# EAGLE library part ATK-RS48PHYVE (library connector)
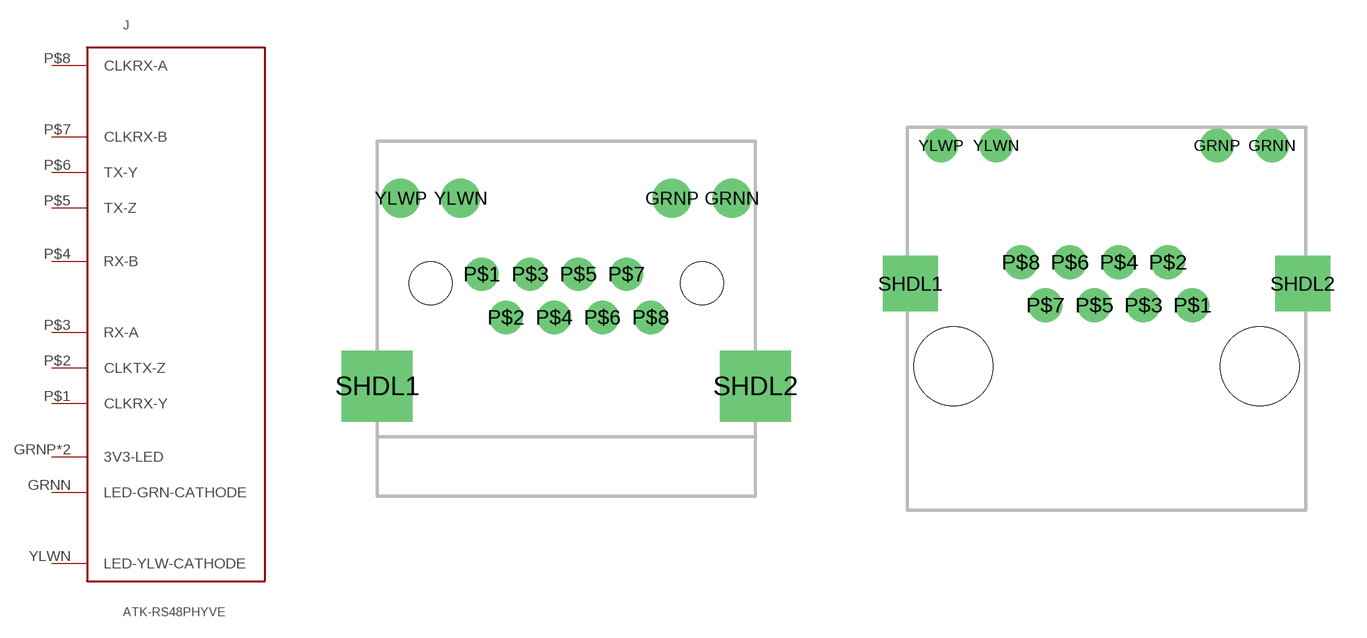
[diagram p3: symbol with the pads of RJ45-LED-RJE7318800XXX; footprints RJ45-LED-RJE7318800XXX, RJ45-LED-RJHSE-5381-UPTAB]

Designator prefix J

## ATK-RS48PHYVERJ45LED  [RJ45-LED-RJE7318800XXX]
GRNN  LED-GRN-CATHODE
GRNP  3V3-LED
P$1  CLKRX-Y
P$2  CLKTX-Z
P$3  RX-A
P$4  RX-B
P$5  TX-Z
P$6  TX-Y
P$7  CLKRX-B
P$8  CLKRX-A
YLWN  LED-YLW-CATHODE
YLWP  3V3-LED

## ATK-RS48PHYVERJ45LEDTABUP  [RJ45-LED-RJHSE-5381-UPTAB]
Pads as for RJ45-LED-RJE7318800XXX

## ATK-RS48PHYVERJ45TABUPSMD  [RJ45-LED-SMD-RJWURTH-634008137521]
Pads as for RJ45-LED-RJE7318800XXX

## Footprint RJ45-LED-RJE7318800XXX (pad centres in mm)
drill 1.1: GRNN 7.01,3.6; GRNP 4.47,3.6; YLWN -4.47,3.6; YLWP -7.01,3.6
drill 0.9: P$1 -3.57,0.38; P$2 -2.55,-1.45; P$3 -1.53,0.38; P$4 -0.51,-1.45; P$5 0.51,0.38; P$6 1.53,-1.45; P$7 2.55,0.38; P$8 3.57,-1.45
drill 2 square: SHDL1 -8,-4.35; SHDL2 8,-4.35
hole 1.8 at -5.74,0
hole 1.8 at 5.74,0

## Footprint RJ45-LED-RJHSE-5381-UPTAB (pad centres in mm)
drill 0.889: GRNN 6.858,6.604; GRNP 4.572,6.604; YLWN -4.572,6.604; YLWP -6.858,6.604
drill 0.9: P$1 3.556,0; P$2 2.54,1.778; P$3 1.524,0; P$4 0.508,1.778; P$5 -0.508,0; P$6 -1.524,1.778; P$7 -2.54,0; P$8 -3.556,1.778
drill 1.524 square: SHDL1 -8.128,0.889; SHDL2 8.128,0.889
hole 3.251 at -6.35,-2.54
hole 3.251 at 6.35,-2.54

## Footprint RJ45-LED-SMD-RJWURTH-634008137521 (pad centres in mm)
smd 0.8 x 3.05: GRNN 6.98,10.8; GRNP 5.71,10.8; YLWN -5.71,10.8; YLWP -6.98,10.8
smd 0.6 x 4.5: P$1 3.57,9.76; P$2 2.55,9.76; P$3 1.53,9.76; P$4 0.51,9.76; P$5 -0.51,9.76; P$6 -1.53,9.76; P$7 -2.55,9.76; P$8 -3.57,9.76
smd 1.2 x 1.8: P$9 -4.9,4.4; P$10 4.9,4.4
smd 2.5 x 4: P$13 -8.65,0; P$14 8.65,0
hole 3.25 at -6.35,0
hole 3.25 at 6.35,0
